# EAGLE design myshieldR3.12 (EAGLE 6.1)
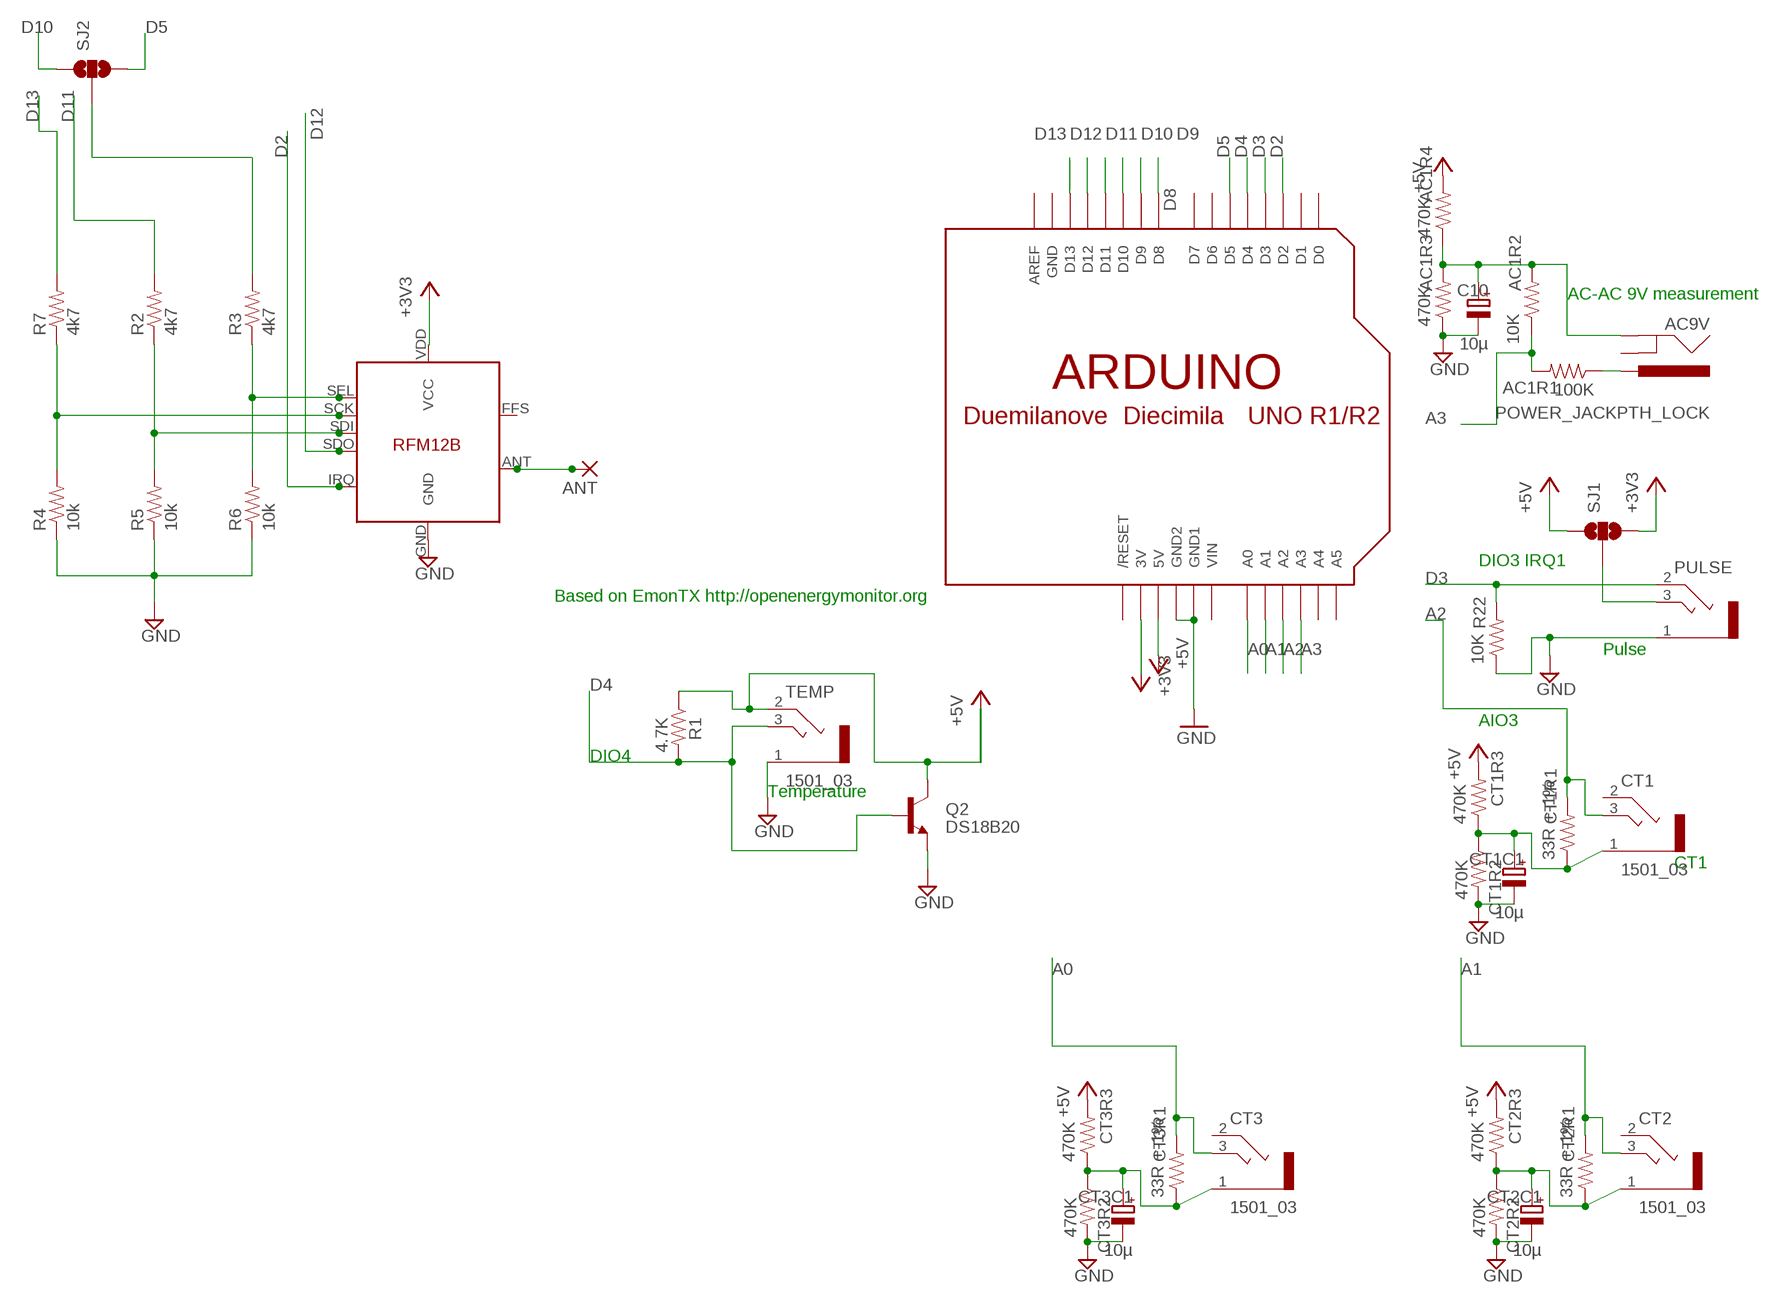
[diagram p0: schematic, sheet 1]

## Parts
AC1R1  100K  RESISTORAXIAL-0.3  [AXIAL-0.3]
AC1R2  10K  RESISTORAXIAL-0.3  [AXIAL-0.3]
AC1R3  470K  RESISTORAXIAL-0.3  [AXIAL-0.3]
AC1R4  470K  RESISTORAXIAL-0.3  [AXIAL-0.3]
AC9V  POWER_JACKPTH_LOCK  [POWER_JACK_PTH_LOCK]
ANT  1,6/0,8  [1,6/0,8]
C10  10µ  CPOL-EUE1.8-4  [E1,8-4]
CT1  1501_03  [1501_03]
CT1C1  10µ  CPOL-EUE1.8-4  [E1,8-4]
CT1R1  33R +-1%  RESISTORAXIAL-0.3  [AXIAL-0.3]
CT1R2  470K  RESISTORAXIAL-0.3  [AXIAL-0.3]
CT1R3  470K  RESISTORAXIAL-0.3  [AXIAL-0.3]
CT2  1501_03  [1501_03]
CT2C1  10µ  CPOL-EUE1.8-4  [E1,8-4]
CT2R1  33R +-1%  RESISTORAXIAL-0.3  [AXIAL-0.3]
CT2R2  470K  RESISTORAXIAL-0.3  [AXIAL-0.3]
CT2R3  470K  RESISTORAXIAL-0.3  [AXIAL-0.3]
CT3  1501_03  [1501_03]
CT3C1  10µ  CPOL-EUE1.8-4  [E1,8-4]
CT3R1  33R +-1%  RESISTORAXIAL-0.3  [AXIAL-0.3]
CT3R2  470K  RESISTORAXIAL-0.3  [AXIAL-0.3]
CT3R3  470K  RESISTORAXIAL-0.3  [AXIAL-0.3]
PULSE  1501_03  [1501_03]
Q2  DS18B20  TRANSISTOR_NPNTO92  [TO-92]
R1  4.7K  RESISTORAXIAL-0.3  [AXIAL-0.3]
R2  4k7  RESISTORAXIAL-0.3  [AXIAL-0.3]
R3  4k7  RESISTORAXIAL-0.3  [AXIAL-0.3]
R4  10k  RESISTORAXIAL-0.3  [AXIAL-0.3]
R5  10k  RESISTORAXIAL-0.3  [AXIAL-0.3]
R6  10k  RESISTORAXIAL-0.3  [AXIAL-0.3]
R7  4k7  RESISTORAXIAL-0.3  [AXIAL-0.3]
R22  10K  RESISTORAXIAL-0.3  [AXIAL-0.3]
SJ1  SOLDERJUMPER_2WAY-OLDS  [SJ_3]
SJ2  SOLDERJUMPER_2WAY-OLDS  [SJ_3]
TEMP  1501_03  [1501_03]
U$1  ARDUINO-NOHOLE  [ARDUINO-NOHOLE]
U$3  RFM12B  [RFM12B]

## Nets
+3V3 [power]: SJ1.3 U$1.3V U$3.VDD(VCC)
+5V [power]: AC1R4.P$2 CT1R3.P$2 CT2R3.P$2 CT3R3.P$2 Q2.3(C) R1.P$1 SJ1.1 TEMP.2 U$1.5V
A0: CT3.3 CT3R1.P$2 U$1.A0
A1: CT2.3 CT2R1.P$2 U$1.A1
A2: CT1.3 CT1R1.P$2 U$1.A2
A3: AC1R1.P$2 AC1R2.P$1 U$1.A3
D2: U$1.D2 U$3.IRQ
D3: PULSE.2 R22.P$2 U$1.D3
D4: Q2.2(B) R1.P$2 TEMP.3 U$1.D4
D5: SJ2.3 U$1.D5
D8: U$1.D8
D9: U$1.D9
D10: SJ2.1 U$1.D10
D11: R2.P$2 U$1.D11
D12: U$1.D12 U$3.SDO
D13: R7.P$2 U$1.D13
GND [power]: AC1R3.P$1 C10.- CT1C1.- CT1R2.P$2 CT2C1.- CT2R2.P$2 CT3C1.- CT3R2.P$2 PULSE.1 Q2.1(E) R4.P$1 R5.P$1 R6.P$1 R22.P$1 TEMP.1 U$1.GND1 U$1.GND2 U$3.GND
N$1: ANT.1(P) U$3.ANT
N$2: R4.P$2 R7.P$1 U$3.SCK
N$4: R2.P$1 R5.P$2 U$3.SDI
N$5: R3.P$1 R6.P$2 U$3.SEL
N$6: CT2.1 CT2C1.+ CT2R1.P$1 CT2R2.P$1 CT2R3.P$1
N$9: R3.P$2 SJ2.2
N$10: CT3.1 CT3C1.+ CT3R1.P$1 CT3R2.P$1 CT3R3.P$1
N$14 [power]: PULSE.3 SJ1.2
N$16 [power]: AC1R2.P$2 AC1R3.P$2 AC1R4.P$1 AC9V.GND C10.+
N$17: CT1.1 CT1C1.+ CT1R1.P$1 CT1R2.P$1 CT1R3.P$1
N$21 [power]: AC1R1.P$1 AC9V.PWR
Unconnected: AC9V.GNDBREAK CT1.2 CT2.2 CT3.2 U$1.A4 U$1.A5 U$1.AREF U$1.D0 U$1.D1 U$1.D6 U$1.D7 U$1.RESET(/RESET) U$3.FFS

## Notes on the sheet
- AC-AC 9V measurement
- DIO3 IRQ1
- Based on EmonTX http://openenergymonitor.org
- Pulse
- AIO3
- DIO4
- Temperature
- CT1

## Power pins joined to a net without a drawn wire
GND: U$1.GND
VIN: U$1.VIN

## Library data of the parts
AC1R1-AC1R4 CT1R1-CT1R3 CT2R1-CT2R3 CT3R1-CT3R3 R1-R7 R22 = SparkFun:RESISTOR: Resistor
AC9V = SparkFun:POWER_JACK: Power Jack This is the standard 5.5mm barrel jack for power. The PTH is the most common, proven, reliable, footprint. All others are experimental. The Slot footprint only works if the mill layer is transmitted to the PCB fab house so be warned. Spark Fun Electronics SKU : PRT-00119. Mating wall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
ANT = JeeLabs:1,6/0,8: THROUGH-HOLE PAD
C10 CT1C1 CT2C1 CT3C1 = resistor:CPOL-EU: POLARIZED CAPACITOR, European symbol
CT1-CT3 PULSE TEMP = con-lumberg:1501_03: Klinkensteckverbinder nach JISC 6560, 2,5 mm Jack connectors according to JISC 6560, 2.5 mm Source: http://www.lumberg.com/Produkte/PDFs/1501_03.pdf; OC_FARNELL: 1200127; OC_NEWARK: unknown
Q2 = SparkFun:TRANSISTOR_NPN: Transistor NPN BJT configuration in SOT23 package. MMBT2222 is the common NPN we use. Double check BCE configuration again layout.
SJ1 SJ2 = SparkFun:SOLDERJUMPER_2WAY-OLD: Solder Jumper 2 way solder jumper
U$1 = adafruit:ARDUINO: Arduino Diecimila/Duemilanove Make a shield with ease, this package has all the named pins as well as the two mounting drill holes and an outline of the USB and DC power connector. The outline is on the DIMENSION layer, so if your board house uses it they will cut the outline to match.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
U$3 = JeeLabs:RFM12B

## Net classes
0 default: width 0.203 mm, drill 0.6 mm, clearance 0.203 mm
1 power: width 0.381 mm, drill 0.6 mm, clearance 0.254 mm

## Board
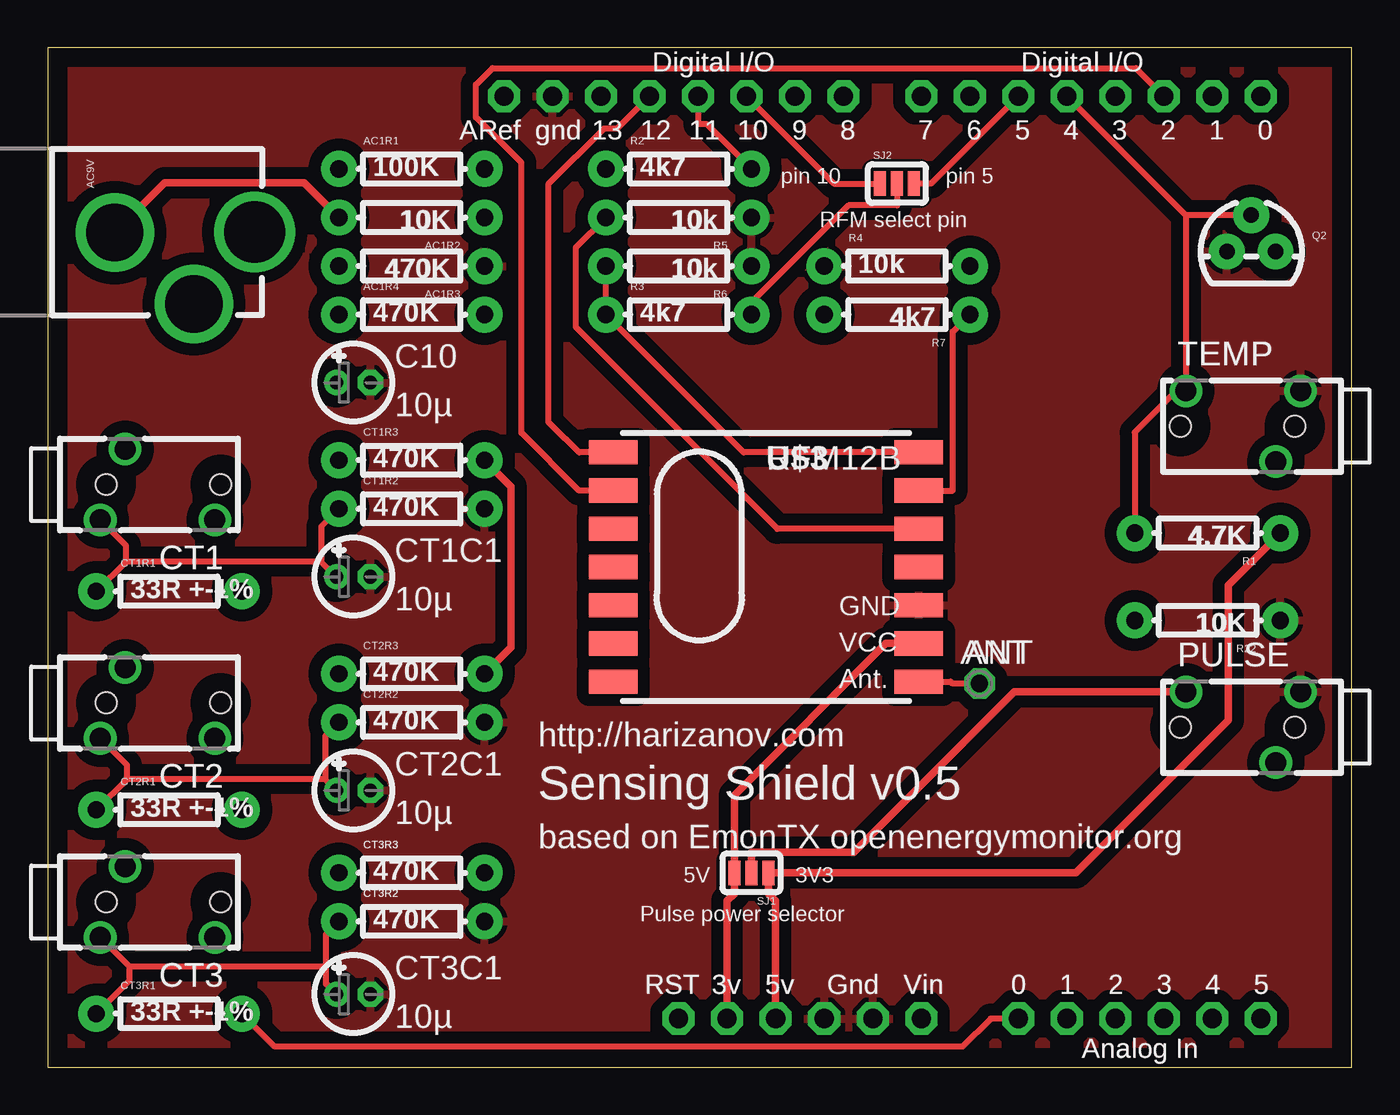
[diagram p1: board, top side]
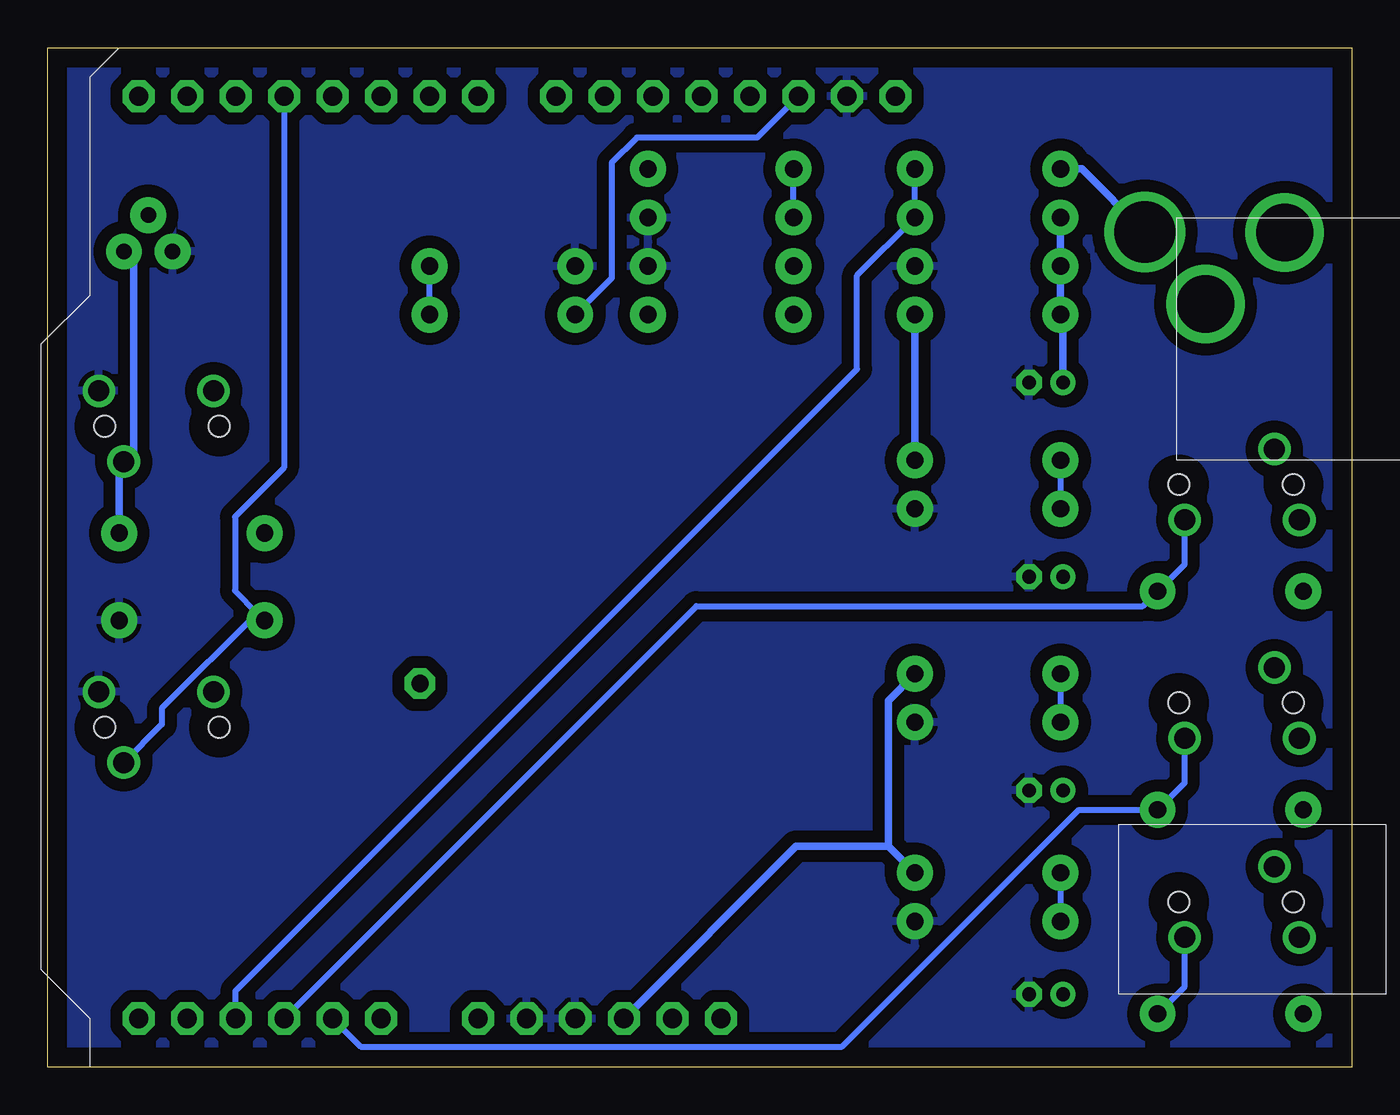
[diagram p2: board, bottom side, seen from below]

Size 68.25 x 53.33 mm. Coordinates in mm from the lower left corner, seen from the top.
Outline: 0,0 68.25,0 68.25,53.33 0,53.33 0,0
Copper layers (1*16): Top 0.035mm / dielectric 1.5mm / Bottom 0.035mm
Design rules: minimum track width 12mil, minimum drill 24mil, track to track 25mil, track to pad 18mil, pad to pad 20mil, via to via 20mil, smd to smd 20mil, copper to edge 40mil, drill to drill 12mil, minimum pad ring 12mil, minimum via ring 12mil, stop-mask expansion 4mil, vias tented up to drill 0mil, thermal gap 10mil

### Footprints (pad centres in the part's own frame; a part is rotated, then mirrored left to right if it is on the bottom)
AXIAL-0.3 = drill 0.9 pad 1.88: P$1 -3.81,0; P$2 3.81,0
POWER_JACK_PTH_LOCK = drill 2.997 pad 4.115: GND 0.025,6.557; GNDBREAK 3.762,10.7 | drill 3.2 pad 4.115: PWR 0,13.878
1,6/0,8 = drill 0.9 pad 1.6 octagon: 1 0,0
E1,8-4 = drill 0.711 pad 1.168: + -0.889,0 | drill 0.711 pad 1.168 octagon: - 0.889,0
1501_03 = drill 1.1 pad 1.7: 1 -1.85,0.3; 2 1.85,-1; 3 -1.85,-5.7 | hole 1.1: 0,0; 0,-6
TO-92 = drill 0.813 pad 1.88: 1 -1.27,0; 2 0,1.905; 3 1.27,0
SJ_3 = smd 0.635 x 1.27: 1 -0.889,0; 2 0,0; 3 0.889,0
ARDUINO-NOHOLE = drill 1 pad 1.676 octagon: 3V 35.56,2.54; 5V 38.1,2.54; A0 50.8,2.54; A1 53.34,2.54; A2 55.88,2.54; A3 58.42,2.54; A4 60.96,2.54; A5 63.5,2.54; AREF 23.876,50.8; D0 63.5,50.8; D1 60.96,50.8; D2 58.42,50.8; D3 55.88,50.8; D4 53.34,50.8; D5 50.8,50.8; D6 48.26,50.8; D7 45.72,50.8; D8 41.656,50.8; D9 39.116,50.8; D10 36.576,50.8; D11 34.036,50.8; D12 31.496,50.8; D13 28.956,50.8; GND 26.416,50.8; GND1 43.18,2.54; GND2 40.64,2.54; RESET 33.02,2.54; VIN 45.72,2.54
RFM12B = smd 2.54 x 1.27: ANT 8,-6; FFS -8,2; GND 8,-2; IRQ -8,4; P$8 -8,0; P$9 -8,-2; P$10 -8,-4; P$12 -8,-6; P$16 8,0; SCK 8,4; SDI 8,2; SDO -8,6; SEL 8,6; VDD 8,-4

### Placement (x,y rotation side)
AC1R1  19.05,46.99 0 top
AC1R2  19.05,44.45 180 top
AC1R3  19.05,41.91 180 top
AC1R4  19.05,39.37 0 top
AC9V  -3.05,43.69 270 top
ANT  48.77,20.07 0 top
C10  16,35.81 0 top
CT1  3.05,30.48 90 top
CT1C1  16,25.65 0 top
CT1R1  6.35,24.89 0 top
CT1R2  19.05,29.21 0 top
CT1R3  19.05,31.75 0 top
CT2  3.05,19.05 90 top
CT2C1  16,14.48 0 top
CT2R1  6.35,13.46 0 top
CT2R2  19.05,18.03 0 top
CT2R3  19.05,20.57 0 top
CT3  3.05,8.64 90 top
CT3C1  16,3.81 0 top
CT3R1  6.35,2.79 0 top
CT3R2  19.05,7.62 0 top
CT3R3  19.05,10.16 0 top
PULSE  65.28,17.78 270 top
Q2  62.99,42.67 0 top
R1  60.71,27.94 180 top
R2  33.02,46.99 0 top
R3  33.02,39.37 0 top
R4  44.45,41.91 0 top
R5  33.02,44.45 180 top
R6  33.02,41.91 180 top
R7  44.45,39.37 180 top
R22  60.71,23.37 180 top
SJ1  36.83,10.16 180 top
SJ2  44.45,46.23 0 top
TEMP  65.28,33.53 270 top
U$1  0,0 0 top
U$3  37.59,26.16 0 top

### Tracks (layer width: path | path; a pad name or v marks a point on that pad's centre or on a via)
+3V3
  Top 0.381: U$1.3V 35.56,3.82 35.56,8.7 35.94,9.08 SJ1.3 35.94,14.23 43.88,22.16 U$3.VDD
+5V
  Top 0.381: U$1.5V 38.1,8.7 37.72,9.08 SJ1.1 53.81,10.16 61.78,18.13 61.78,25.2 R1.P$1 | CT2R3.P$2 24.26,21.97 24.26,30.35 CT1R3.P$2
  Bottom 0.381: 24.26,11.56 24.26,19.17 CT2R3.P$2 | CT3R3.P$2 24.26,11.56 | U$1.5V 29.08,11.56 24.26,11.56 | Q2.3 63.76,42.17 63.76,32.2 TEMP.2 64.52,31.44 R1.P$1 | CT1R3.P$2 AC1R4.P$2
A0
  Top 0.305: U$1.A0 49.35,2.54 47.88,1.07 11.88,1.07 CT3R1.P$2
  Bottom 0.305: CT3R1.P$2 8.75,4.21 CT3.3
A1
  Bottom 0.305: U$1.A1 51.87,1.07 26.67,1.07 14.28,13.46 CT2R1.P$2 8.75,14.87 CT2.3
A2
  Bottom 0.305: U$1.A2 34.31,24.11 10.94,24.11 CT1R1.P$2 8.75,26.3 CT1.3
A3
  Bottom 0.305: U$1.A3 58.42,3.99 25.89,36.52 25.89,41.42 AC1R2.P$1 AC1R1.P$2
D2
  Top 0.305: U$3.IRQ 27.81,30.16 24.79,33.18 24.79,47.32 22.42,49.69 22.42,51.4 23.28,52.26 56.96,52.26 U$1.D2
D3
  Bottom 0.305: 57.28,23.76 R22.P$2 | U$1.D3 55.88,31.36 58.45,28.79 58.45,24.92 57.28,23.76 | 57.28,23.76 62.28,18.76 62.28,17.93 PULSE.2
D4
  Top 0.305: R1.P$2 56.9,33.21 59.06,35.38 TEMP.3 59.58,44.58 | 59.58,44.58 59.56,44.58 U$1.D4 | Q2.2 59.58,44.58
D5
  Top 0.305: U$1.D5 46.23,46.23 SJ2.3
D10
  Top 0.305: U$1.D10 41.15,46.23 SJ2.1
D11
  Top 0.305: U$1.D11 34.04,49.35 34.47,49.35 R2.P$2
D12
  Top 0.305: U$1.D12 29.79,49.09 29.11,49.09 26.19,46.18 26.19,33.76 27.07,32.88 27.1,32.88 | 27.1,32.88 | 27.1,32.88 27.81,32.16 U$3.SDO
D13
  Bottom 0.305: U$1.D13 31.13,48.63 37.42,48.63 38.73,47.31 38.73,41.27 R7.P$2
GND
  pour Bottom (isolate 0.305): 0,53.34 68.58,53.34 68.58,52.07 68.58,0 0,0
  pour Top (isolate 0.305): 0,53.34 68.58,53.34 68.58,0 0,0
N$1
  Top 0.305: ANT.1 47.36,20.07 47.26,20.16 U$3.ANT
N$2
  Top 0.305: U$3.SCK 47.37,30.16 47.37,38.48 R7.P$1
  Bottom 0.305: R7.P$1 R4.P$2
N$4
  Top 0.305: U$3.SDI 38.19,28.16 27.65,38.71 27.65,42.89 R5.P$2
  Bottom 0.305: R5.P$2 R2.P$1
N$5
  Top 0.305: R6.P$2 R3.P$1 36.42,32.16 U$3.SEL
N$6
  Top 0.305: 14.52,15.07 4.15,15.07 | CT2C1.+ 14.52,15.07 | CT2R2.P$1 14.52,17.32 14.52,15.07 | 4.15,15.07 CT2R1.P$1 | 4.15,15.07 4.15,15.8 CT2.1
  Bottom 0.305: CT2R3.P$1 CT2R2.P$1
N$9
  Top 0.305: SJ2.2 44.45,45.08 41.91,45.08 36.83,40.01 R3.P$2
N$10
  Top 0.305: 4.28,5.25 CT3.1 | 14.57,5.25 4.28,5.25 | CT3R1.P$1 4.28,4.54 4.28,5.25 | 14.57,5.25 14.57,6.95 CT3R2.P$1 | CT3C1.+ 14.57,4.36 14.57,5.25
  Bottom 0.305: CT3R3.P$1 CT3R2.P$1
N$14
  Top 0.381: SJ1.2 36.83,11.24 42.2,11.24 50.59,19.63 PULSE.3
N$16
  Top 0.381: AC1R2.P$2 13.42,46.27 6.11,46.27 AC9V.GND
  Bottom 0.381: AC1R2.P$2 AC1R3.P$2 AC1R4.P$1 15.11,39.24 C10.+
N$17
  Top 0.305: 14.32,26.45 4.1,26.45 | CT1C1.+ 14.32,26.45 | CT1R2.P$1 14.32,28.29 14.32,26.45 | 4.1,26.45 CT1R1.P$1 | 4.1,26.45 4.1,27.28 CT1.1
  Bottom 0.305: CT1R3.P$1 CT1R2.P$1
N$21
  Bottom 0.381: AC9V.PWR 14.13,46.99 AC1R1.P$1

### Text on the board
_tsilk: Digital I/O | Digital I/O | ARef | gnd | 13 | 12 | 11 | 10 | 9 | 8 | 7 | 6 | 5 | 4 | 3 | 2 | 1 | 0 | 100K | 4k7 | pin 10 | pin 5 | 10K | 10k | RFM select pin | 470K | 10k | 10k | 470K | 4k7 | 4k7 | TEMP | 10µ | 470K | RFM12B | 470K | 4.7K | CT1 | 33R +-1% | 10µ | 10K | ANT | PULSE | 470K | 470K | CT2 | http://harizanov.com | Sensing Shield v0.5 | 33R +-1% | 10µ | CT3R3 | based on EmonTX openenergymonitor.org | CT3R2 | 470K | 5V | 3V3 | 470K | Pulse power selector | CT3 | RST | 3v | 5v | Gnd | Vin | 0 | 1 | 2 | 3 | 4 | 5 | 33R +-1% | 10µ | Analog In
